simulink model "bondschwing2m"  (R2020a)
settings: Solver=ode45  StartTime=0.0  StopTime=40  RelTol=1e-3  EnableMultiTasking=on
undefined symbols (not defined in the file or in its folder): Display, Int, libbondgraph
libraries: libbondgraph x12

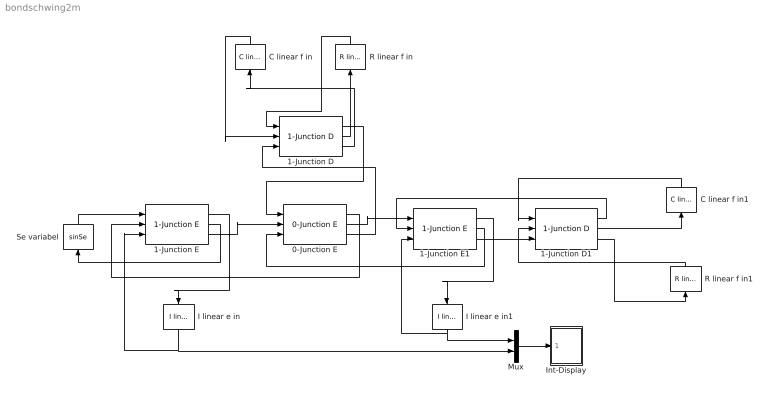
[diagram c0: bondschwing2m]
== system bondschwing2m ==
  0-Junction E : libbondgraph/0-Junction E
  1-Junction D : libbondgraph/1-Junction D
  1-Junction D1 : libbondgraph/1-Junction D
  1-Junction E : libbondgraph/1-Junction E
  1-Junction E1 : libbondgraph/1-Junction E
  C linear f in : libbondgraph/C linear f in  C=1
  C linear f in1 : libbondgraph/C linear f in  C=1
  I linear e in : libbondgraph/I linear e in  I=1
  I linear e in1 : libbondgraph/I linear e in  I=1
  Int-Display : Subsystem  AncestorBlock=libbondgraph/Int-Display
  Mux : Mux  Inputs=2
  R linear f in : libbondgraph/R linear f in  R=1
  R linear f in1 : libbondgraph/R linear f in  R=1
  Se variabel : libbondgraph/sinSe  amplitude=1  frequency=3
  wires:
  Se variabel/1 -> 1-Junction E/1
  1-Junction E/2 -> Se variabel/1
  1-Junction E/1 -> I linear e in/1
  I linear e in/1 -> 1-Junction E/3, Mux/2
  1-Junction E/3 -> 0-Junction E/2
  0-Junction E/1 -> 1-Junction E/2
  0-Junction E/3 -> 1-Junction D/3
  1-Junction D/1 -> 0-Junction E/1
  0-Junction E/2 -> 1-Junction E1/1
  1-Junction E1/2 -> 0-Junction E/3
  1-Junction D/2 -> R linear f in/1
  R linear f in/1 -> 1-Junction D/1
  1-Junction D/3 -> C linear f in/1
  C linear f in/1 -> 1-Junction D/2
  1-Junction E1/1 -> I linear e in1/1
  I linear e in1/1 -> 1-Junction E1/3, Mux/1
  1-Junction E1/3 -> 1-Junction D1/3
  1-Junction D1/1 -> 1-Junction E1/2
  1-Junction D1/2 -> C linear f in1/1
  C linear f in1/1 -> 1-Junction D1/1
  1-Junction D1/3 -> R linear f in1/1
  R linear f in1/1 -> 1-Junction D1/2
  Mux/1 -> Int-Display/1(In1)

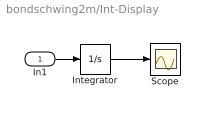
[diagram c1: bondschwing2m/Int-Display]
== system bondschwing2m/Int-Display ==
  In1 : Inport
  Integrator : Integrator
  Scope : Scope
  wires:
  Integrator/1 -> Scope/1
  In1/1 -> Integrator/1
